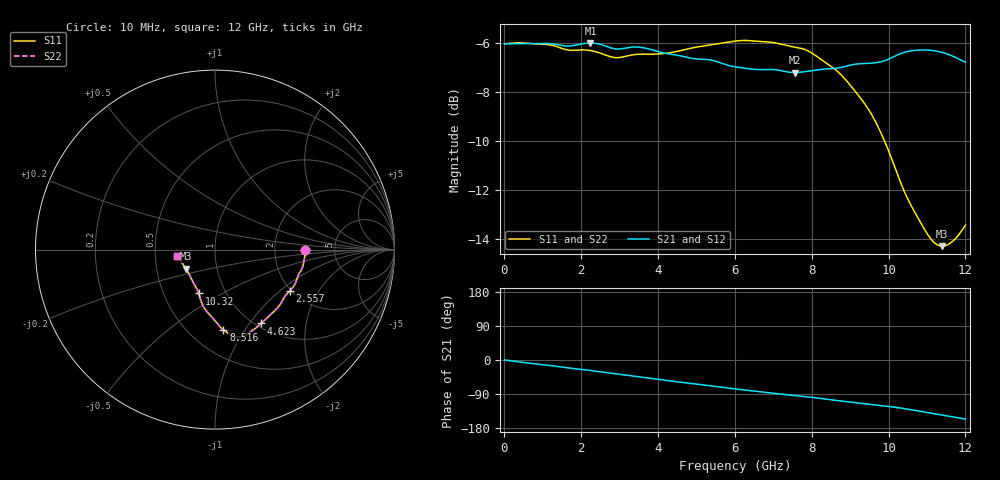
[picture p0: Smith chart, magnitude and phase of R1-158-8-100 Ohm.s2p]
!version-1
!date-10.2020
!Series
#GHZ	S	RI	R	50.0
!FREQ.GHZ	S11RE	S11IM	S21RE	S21IM	S12RE	S12IM	S22RE	S22IM
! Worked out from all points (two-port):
!   500 points, 10 MHz to 12 GHz, reference 50 ohm
!   highest |S21| = -5.99 dB at 2.245 GHz (marker M1); lowest = -7.2 dB at 7.555 GHz (marker M2)
!   |S21| within 3 dB of the highest: start of sweep to end of sweep
!   lowest |S11| = -14.3 dB at 11.4 GHz (marker M3), VSWR 1.48, Z = 35.3 - j7.74 ohm
!   |S11| at or under -10 dB: 9.9 GHz to end of sweep
!   |S22| runs from -14.3 to -5.9 dB; largest |S21 - S12| = 0
!   S11 on the Smith chart (normalised r, x): 10 MHz: 3.00, +0.00; 2.557 GHz: 1.98, -1.17; 4.623 GHz: 1.06, -1.14; 8.516 GHz: 0.72, -0.81; 10.32 GHz: 0.75, -0.39; 12 GHz: 0.65, -0.05
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0.01  0.5 0  0.5 0  0.5 0  0.5 0
1.09126  0.4903 -0.0897  0.4872 -0.1159  0.4872 -0.1159  0.4903 -0.0897
2.02836  0.4523 -0.1773  0.453 -0.2112  0.453 -0.2112  0.4523 -0.1773
2.24461  0.4415 -0.1992  0.4438 -0.2337  0.4438 -0.2337  0.4415 -0.1992
2.55697  0.4182 -0.2289  0.421 -0.2646  0.421 -0.2646  0.4182 -0.2289
2.91739  0.3903 -0.259  0.3913 -0.2914  0.3913 -0.2914  0.3903 -0.259
3.44601  0.3565 -0.315  0.3572 -0.3391  0.3572 -0.3391  0.3565 -0.315
4.02269  0.3061 -0.3655  0.3012 -0.3759  0.3012 -0.3759  0.3061 -0.3655
4.62339  0.257 -0.4112  0.2419 -0.4051  0.2419 -0.4051  0.257 -0.4112
5.39228  0.203 -0.4544  0.1708 -0.4303  0.1708 -0.4303  0.203 -0.4544
6.01701  0.1667 -0.4782  0.1055 -0.436  0.1055 -0.436  0.1667 -0.4782
6.90605  0.1278 -0.4874  0.0265 -0.4426  0.0265 -0.4426  0.1278 -0.4874
7.55481  0.1011 -0.4819  -0.0297 -0.4359  -0.0297 -0.4359  0.1011 -0.4819
8.01134  0.0779 -0.472  -0.0668 -0.4357  -0.0668 -0.4357  0.0779 -0.472
8.51593  0.0465 -0.4465  -0.1174 -0.4292  -0.1174 -0.4292  0.0465 -0.4465
9.429  -0.0228 -0.3718  -0.2006 -0.4094  -0.2006 -0.4094  -0.0228 -0.3718
10.0057  -0.076 -0.2921  -0.2509 -0.392  -0.2509 -0.392  -0.076 -0.2921
10.318  -0.0901 -0.2441  -0.2862 -0.3825  -0.2862 -0.3825  -0.0901 -0.2441
11.0148  -0.1356 -0.153  -0.365 -0.3201  -0.365 -0.3201  -0.1356 -0.153
11.3993  -0.1621 -0.1053  -0.3961 -0.2712  -0.3961 -0.2712  -0.1621 -0.1053
11.6636  -0.1833 -0.074  -0.4098 -0.2343  -0.4098 -0.2343  -0.1833 -0.074
12  -0.2107 -0.0337  -0.4187 -0.1872  -0.4187 -0.1872  -0.2107 -0.0337
